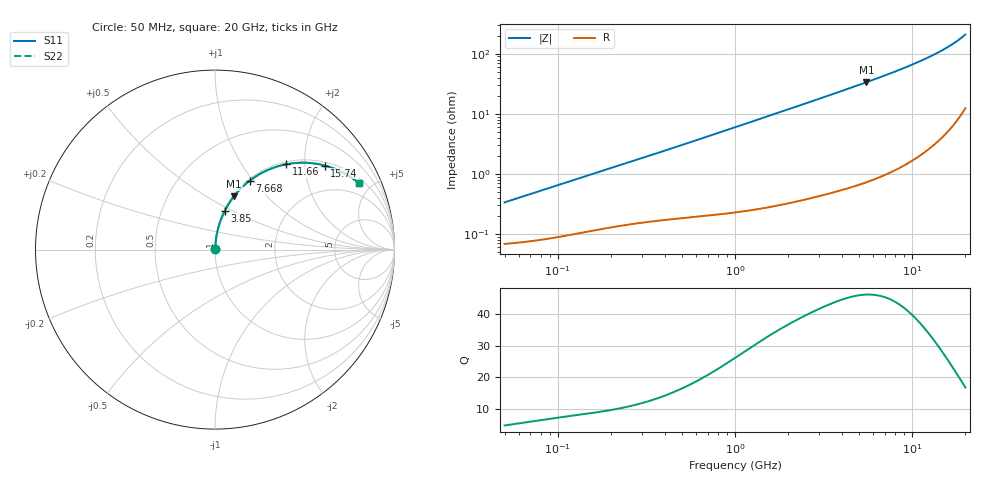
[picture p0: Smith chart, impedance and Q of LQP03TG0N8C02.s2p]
!Murata Part Number: LQP03TG0N8C02
!These Parameters are Measured in Series Mode Connection
!  o--[Z]--o
!Port1  Port2
!  o-------o
!Freq. Start=50[MHz] Stop=20[GHz], 401[Steps]
# Hz S RI R 50
!Freq.(Hz) S11(Real) S11(Imag) S21(Real) S21(Imag) S12(Real) S12(Imag) S22(Real) S22(Imag)
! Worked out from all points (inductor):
!   401 points, 50 MHz to 20 GHz, reference 50 ohm
!   read as one part in series: L = 1.05 nH near 51.52 MHz
!   highest Q = 46.1 at 5.516 GHz (marker M1), where L = 967 pH
!   S11 on the Smith chart (normalised r, x): 50 MHz: 1.00, +0.01; 3.85 GHz: 1.01, +0.46; 7.668 GHz: 1.02, +0.96; 11.66 GHz: 1.05, +1.61; 15.74 GHz: 1.10, +2.53; 20 GHz: 1.25, +4.18
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5e7  0.000697 0.00329  0.9993 -0.00329  0.9993 -0.00329  0.000697 0.00329
5.152053e7  0.000703 0.00339  0.9993 -0.00339  0.9993 -0.00339  0.000703 0.00339
1.364002e8  0.00113 0.00871  0.9989 -0.00871  0.9989 -0.00871  0.00113 0.00871
3.721004e8  0.00218 0.0226  0.9978 -0.0226  0.9978 -0.0226  0.00218 0.0226
6.380365e8  0.00343 0.0381  0.9966 -0.0381  0.9966 -0.0381  0.00343 0.0381
1e9  0.00581 0.0592  0.9942 -0.0592  0.9942 -0.0592  0.00581 0.0592
1.714689e9  0.0132 0.1004  0.9868 -0.1004  0.9868 -0.1004  0.0132 0.1004
2.728004e9  0.0294 0.157  0.9706 -0.157  0.9706 -0.157  0.0294 0.157
3.850025e9  0.0549 0.2166  0.9451 -0.2166  0.9451 -0.2166  0.0549 0.2166
4.677679e9  0.0784 0.2581  0.9216 -0.2581  0.9216 -0.2581  0.0784 0.2581
5.515528e9  0.1061 0.2974  0.8939 -0.2974  0.8939 -0.2974  0.1061 0.2974
6.406762e9  0.1396 0.3358  0.8604 -0.3358  0.8604 -0.3358  0.1396 0.3358
7.442007e9  0.1831 0.3757  0.8169 -0.3757  0.8169 -0.3757  0.1831 0.3757
7.668323e9  0.1932 0.3837  0.8068 -0.3837  0.8068 -0.3837  0.1932 0.3837
9.457416e9  0.2791 0.4365  0.7209 -0.4365  0.7209 -0.4365  0.2791 0.4365
1.050288e10  0.3332 0.4585  0.6668 -0.4585  0.6668 -0.4585  0.3332 0.4585
1.166392e10  0.3952 0.4751  0.6048 -0.4751  0.6048 -0.4751  0.3952 0.4751
1.375312e10  0.5083 0.4838  0.4917 -0.4838  0.4917 -0.4838  0.5083 0.4838
1.573793e10  0.6119 0.4684  0.3881 -0.4684  0.3881 -0.4684  0.6119 0.4684
1.747767e10  0.6957 0.4379  0.3043 -0.4379  0.3043 -0.4379  0.6957 0.4379
1.940974e10  0.7777 0.3889  0.2223 -0.3889  0.2223 -0.3889  0.7777 0.3889
2e10  0.8001 0.3713  0.1999 -0.3713  0.1999 -0.3713  0.8001 0.3713
